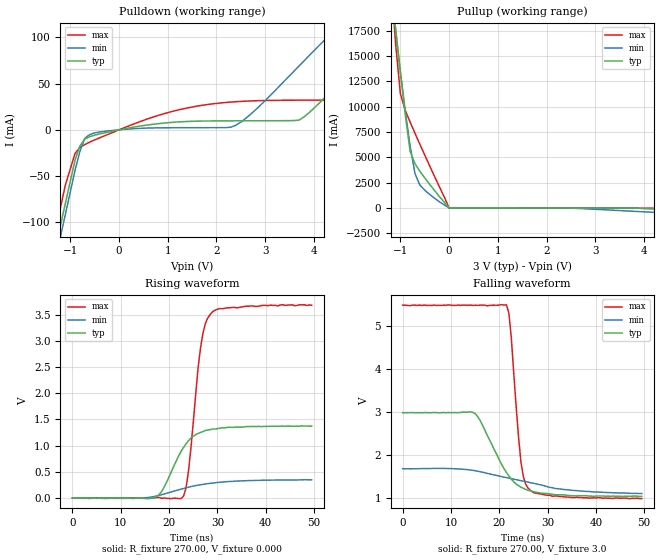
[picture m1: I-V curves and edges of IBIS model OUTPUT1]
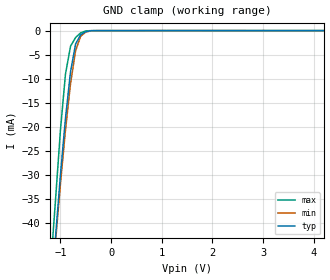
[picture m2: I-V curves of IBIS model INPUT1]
| IBIS file 8025nb.ibs
[IBIS ver]   3.0
[File name]   8025nb.ibs
[File Rev]   1.0
[Date]   Mar 22, 2004
[Source]   This file orginated at SEIKO EPSON QD Div.
[Copyright]   Copyright SEIKO EPSON Corp. 2004
|   Component 8025nb
[Component]   8025nb
[Manufacturer]   SEIKO EPSON
[Package]
| variable   typ   min   max
R_pkg   87m   NA   NA
L_pkg   10nH   NA   NA
C_pkg   206fF   NA   NA
[Pin]  signal_name   model_name   R_pin   L_pin   C_pin
1   FOE   INPUT1
2   VDD   POWER
|3   GND
|4   TEST
5   FOUT   OUTPUT1
|6   SCL   POWER
|7   SDA
|8   /INTB
9   GND   GND
| Models and submodels in the file (2): OUTPUT1 (Output), INPUT1 (Input)
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|10   /INTA
|11   NC
|12
|13
|14   NC
|15   NC
|16   NC
|17   NC
|18   NC
|19   NC
|20   NC
|21   NC
|22   NC
|   Model OUTPUT
[Model]   OUTPUT1
Model_type   Output
Polarity   Non-Inverting
Enable   Active-High
Vmeas =   1.50V
C_comp   1.69pF   1.32pF   1.96pF
[Temperature Range]   25.00   85.00   -40.000
[Voltage Range]   3.0V   1.7V   5.5V
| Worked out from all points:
|   slope of the pulldown table from 0 to 0.45 V, typ, clamps not added: 108 ohm
|   slope of the pullup table from 0 to 0.45 V, typ, clamps not added: 208 ohm
|   rising waveform, R_fixture 270.00, V_fixture 0.000: 20-80 % time 4.72ns typ, 9.66ns min, 2.38ns max; typ from -0.005 V to 1.37 V
|   falling waveform, R_fixture 270.00, V_fixture 3.0: 20-80 % time 5.64ns typ, 14ns min, 1.86ns max; typ from 2.99 V to 1.04 V
[Pulldown]
| voltage   I(typ)   I(min)   I(max)
-5.5V     -1.119A    -1.147A    -1.122A
-1.4V     -150.5mA   -163.5mA   -132.1mA
-1.2V     -103.3mA   -115.5mA   -83.87mA
-900mV    -32.47mA   -43.53mA   -25.45mA
-600mV    -7.38mA    -5.17mA    -13.23mA
2.4V      9.76mA     4.99mA     30.38mA
3.7V      10.61mA    69.14mA    32.04mA
4.5V      49.94mA    111.9mA    32.08mA
5.7V      112.4mA    176mA      32.02mA
6.4V      146.3mA    213.4mA    35.38mA
7.5V      199.5mA    272.1mA    101.8mA
11V       368.9mA    459mA      288.4mA
[Pullup]
| voltage   I(typ)   I(min)   I(max)
-5.5V     242.4A     238.7A     275.5A
-1.2V     22.3A      22.09A     23.22A
-1.1V     17.68A     17.72A     16.3A
-1V       13.31A     13.5A      11.27A
-800mV    5.59A      6.11A      8.48A
-700mV    4.36A      3.39A      7.37A
-600mV    3.62A      2.26A      6.29A
-500mV    2.96A      1.75A      5.22A
0V        20uA       10uA       80uA
3.8V      -19.71mA   -337.3mA   -21.21mA
6.4V      -662.1mA   -983.6mA   -35.23mA
11V       -1.809A    -2.127A    -1.045A
[Ramp]
| variable   typ   min   max
dV/dt_r 0.84/6.5n   0.21/11n   2.23/2.0n
dV/dt_f 1.18/5.5n   0.32/15n   2.71/2.0n
R_load = 300.00
[Rising Waveform]
R_fixture = 270.00
V_fixture = 0.000
| time   V(typ)   V(min)   V(max)
0s        -4.61mV    -9.91mV    -8.75mV
17ns      230uV      23.39mV    -2.66mV
18.5ns    123.3mV    57.23mV    -13.44mV
22.5ns    889.3mV    164mV      -17.97mV
23.5ns    1.03V      188.9mV    180.9mV
24ns      1.09V      200.3mV    489.2mV
26.5ns    1.251V     246.8mV    2.864V
28ns      1.298V     268.8mV    3.447V
30.5ns    1.333V     295.4mV    3.629V
49.5ns    1.374V     342.5mV    3.692V
[Falling Waveform]
R_fixture = 270.00
V_fixture = 3.0
V_fixture_min = 1.7
V_fixture_max = 5.5
| time   V(typ)   V(min)   V(max)
0s        2.991V     1.687V     5.491V
15ns      2.97V      1.641V     5.49V
21.5ns    1.598V     1.48V      5.499V
22ns      1.517V     1.467V     5.301V
22.5ns    1.444V     1.458V     4.732V
23.5ns    1.329V     1.433V     3.135V
24.5ns    1.254V     1.408V     1.833V
25ns      1.233V     1.398V     1.498V
26ns      1.183V     1.377V     1.231V
49.5ns    1.042V     1.109V     991.4mV
|   Model INPUT1
[Model]   INPUT1
Model_type   Input
Polarity   Non-Inverting
C_comp   0.80pF   0.60pF   1.00pF
[Temperature Range]   25.00   85.00   -40.00
[Voltage Range]   3.0V   1.7V   5.50V
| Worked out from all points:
|   GND clamp passes 1 mA (typ) near -0.61 V on its own axis
[GND_clamp]
| voltage   I(typ)   I(min)   I(max)
-5.5V     -661.1mA   -658.8mA   -669.7mA
-1.2V     -57.41mA   -57.36mA   -50.12mA
-1.1V     -43.37mA   -44.35mA   -35.71mA
-1V       -30.11mA   -31.95mA   -20.77mA
-900mV    -18.25mA   -20.7mA    -9.03mA
-800mV    -8.54mA    -11.01mA   -3.24mA
-700mV    -2.78mA    -4.18mA    -1.43mA
-600mV    -850uA     -1.17mA    -470uA
-500mV    -230uA     -310uA     -60uA
-400mV    -30uA      -50uA      0A
-200mV    0A         0A         0A
5.5V      0A         0A         0A
